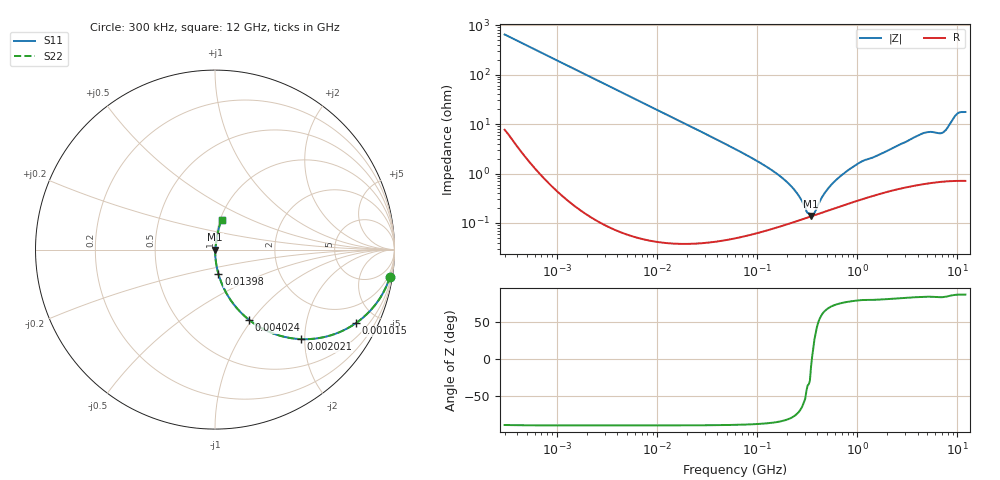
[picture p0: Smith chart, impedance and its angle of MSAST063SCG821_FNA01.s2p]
! MSAST063SCG821_FNA01  S-PARAMETER MODEL  ( General Type )
! Model Generated by TAIYO YUDEN Corporation (http://www.ty-top.com)
! Version 1.0
! TAIYO YUDEN Control No. 160830
! Copyright(c) 2016 TAIYO YUDEN CO.,LTD. All Rights Reserved.
! Product Description (link to TY-COMPAS)
! https://ds.yuden.co.jp/TYCOMPAS/or/detail?pn=MSAST063SCG821JFNA01&u=M
! Products Name : Multilayer Ceramic Capacitors
! Characteristics :
!  Capacitance : 820 pF , Rated Voltage : 25V , TCC : CG / C0G
!  Case Size : 0.6 x 0.3 / 0.024 x 0.012 [mm/inch] , Thickness : 0.3 / 0.012 [mm/inch]
!  (Conditions: Temperature = 25 degC , DC Bias Current/Voltage = 0A / 0V)
! External Node Assignments :
!  1  o---| |---o  2
! GND o---------o GND
! Frequency Range : 0.3MHz  -  12000MHz  [ 401 STEP ]
# MHz S RI R 50
! Freq[MHz].  S11 Real  S11 Imag  S21 Real  S21 Imag  S12 Real  S12 Imag  S22 Real  S22 Imag
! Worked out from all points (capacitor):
!   401 points, 300 kHz to 12 GHz, reference 50 ohm
!   read as one part in series: C = 820 pF near 316.3 kHz
!   lowest |Z| = 138 mohm at 344.7 MHz (marker M1)
!   series resonance near 351.6 MHz, so ESL is about 250 pH
!   S11 on the Smith chart (normalised r, x): 300 kHz: 1, -13; 1.015 MHz: 1.01, -3.83; 2.021 MHz: 1.00, -1.92; 4.024 MHz: 1.00, -0.96; 13.98 MHz: 1.00, -0.28; 12 GHz: 1.01, +0.35
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0.3  0.975 -0.1504  0.025 0.1504  0.025 0.1504  0.975 -0.1504
0.597386  0.9125 -0.2805  0.0875 0.2805  0.0875 0.2805  0.9125 -0.2805
1.014748  0.7848 -0.4098  0.2152 0.4098  0.2152 0.4098  0.7848 -0.4098
1.769972  0.5459 -0.4971  0.4541 0.4971  0.4541 0.4971  0.5459 -0.4971
2.020654  0.4799 -0.4988  0.5201 0.4988  0.5201 0.4988  0.4799 -0.4988
4.023703  0.1891 -0.3908  0.8109 0.3908  0.8109 0.3908  0.1891 -0.3908
10.44266  0.0337 -0.1794  0.9663 0.1794  0.9663 0.1794  0.0337 -0.1794
13.97552  0.0192 -0.1359  0.9808 0.1359  0.9808 0.1359  0.0192 -0.1359
60  0.00147 -0.0313  0.9985 0.0313  0.9985 0.0313  0.00147 -0.0313
187.4445  0.000959 -0.00739  0.999 0.00739  0.999 0.00739  0.000959 -0.00739
244.3004  0.00109 -0.0041  0.9989 0.0041  0.9989 0.0041  0.00109 -0.0041
310.0777  0.00126 -0.00117  0.9987 0.00117  0.9987 0.00117  0.00126 -0.00117
344.7396  0.00136 -0.000245  0.9986 0.000245  0.9986 0.000245  0.00136 -0.000245
353.9943  0.00138 8.75e-05  0.9986 -8.75e-05  0.9986 -8.75e-05  0.00138 8.75e-05
486.4723  0.00174 0.00402  0.9983 -0.00402  0.9983 -0.00402  0.00174 0.00402
668.5285  0.00221 0.00834  0.9978 -0.00834  0.9978 -0.00834  0.00221 0.00834
1076.992  0.00322 0.0167  0.9968 -0.0167  0.9968 -0.0167  0.00322 0.0167
2088.533  0.00523 0.0295  0.9948 -0.0295  0.9948 -0.0295  0.00523 0.0295
4623.766  0.0103 0.0648  0.9897 -0.0648  0.9897 -0.0648  0.0103 0.0648
7064.448  0.0111 0.0651  0.9889 -0.0651  0.9889 -0.0651  0.0111 0.0651
9708.23  0.0298 0.1486  0.9702 -0.1486  0.9702 -0.1486  0.0298 0.1486
12000  0.0362 0.1677  0.9638 -0.1677  0.9638 -0.1677  0.0362 0.1677
